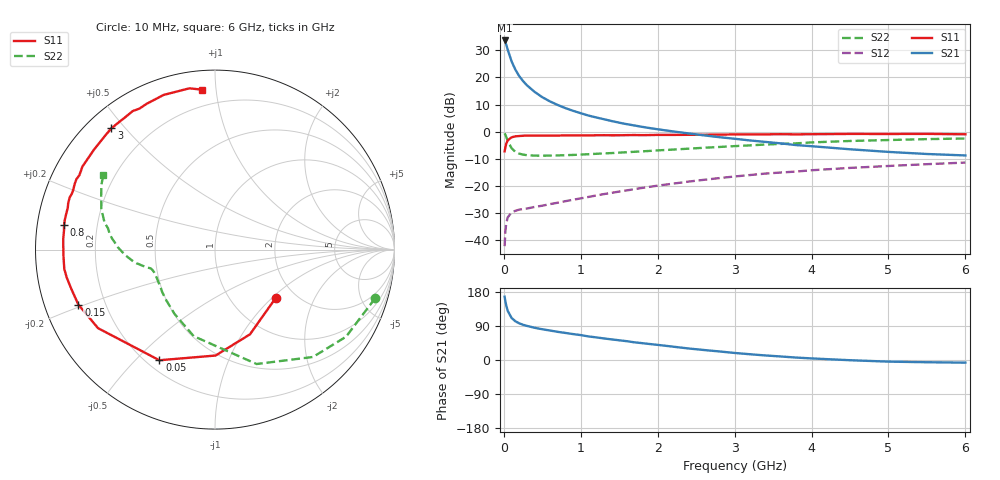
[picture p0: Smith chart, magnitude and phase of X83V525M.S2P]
! SIEMENS Small Signal Semiconductors
! BFP136W
! Si NPN RF Bipolar Junction Transistor in SOT343
! VCE = 3.5 V  IC = 25 mA
! Common Emitter S-Parameters:  September  1994
# GHz  S  MA  R  50
!  f  S11  S21  S12  S22
! GHz  MAG  ANG  MAG  ANG  MAG  ANG  MAG  ANG
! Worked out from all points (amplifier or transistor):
!   40 points, 10 MHz to 6 GHz, reference 50 ohm
!   highest |S21| = 33.7 dB at 10 MHz (marker M1)
!   |S21| within 3 dB of that: start of sweep to 46.27 MHz
!   unconditionally stable (mu >= 1): 831.5 MHz to 2.812 GHz
!   at 200 MHz: K = 0.38, MSG = 24.6 dB, |S12| = -28.8 dB
!   at 1.5 GHz: K = 1.16, MAG = 10.3 dB, |S12| = -22.1 dB
!   at 6 GHz: K = 0.97, MSG = 1.3 dB, |S12| = -11.4 dB
!   S11 on the Smith chart (normalised r, x): 10 MHz: 1.60, -1.05; 50 MHz: 0.25, -0.59; 150 MHz: 0.10, -0.19; 800 MHz: 0.08, +0.08; 3 GHz: 0.07, +0.46; 6 GHz: 0.10, +0.92
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0.01  0.4323 -38.2  48.23 167.0  0.0077 76.1  0.9325 -16.9
0.02  0.5108 -67.6  44.61 155.0  0.0144 67.2  0.8768 -33.6
0.03  0.5902 -89.7  40.99 145.0  0.0198 58.3  0.8099 -47.6
0.05  0.6901 -116.7  32.74 129.9  0.0261 44.4  0.6784 -70.0
0.1  0.785 -146.1  19.94 111.1  0.0323 31.4  0.4968 -103.8
0.15  0.8207 -158.1  13.93 102.2  0.0346 27.7  0.4232 -122.2
0.2  0.8301 -164.8  10.58 96.8  0.0364 26.7  0.3923 -133.6
0.25  0.8407 -169.4  8.576 92.9  0.0374 27.1  0.3776 -141.1
0.3  0.8466 -172.7  7.184 90.0  0.0381 27.9  0.3676 -146.3
0.4  0.8451 -177.9  5.423 85.1  0.0408 30.7  0.3612 -153.0
0.5  0.8457 178.4  4.326 81.1  0.043 33.5  0.3601 -157.1
0.6  0.8477 176.0  3.611 77.8  0.046 36.3  0.3616 -159.5
0.7  0.8478 173.0  3.111 74.3  0.0488 39.3  0.3644 -161.0
0.8  0.852 170.8  2.719 71.4  0.0521 41.6  0.3679 -162.4
1.1  0.8527 164.1  1.982 62.2  0.0624 46.8  0.3837 -164.7
1.6  0.8633 154.9  1.373 49.6  0.0825 51.4  0.4176 -167.8
2.2  0.871 144.5  1.01 35.2  0.1097 52.1  0.4668 -172.6
3  0.8888 130.5  0.74 18.6  0.1489 48.3  0.5408 178.7
3.2  0.8889 127.1  0.688 15.2  0.1582 46.8  0.5585 176.1
4.5  0.908 108.4  0.473 -0.6  0.2144 35.6  0.6732 160.2
5.5  0.9099 99.0  0.387 -5.9  0.2511 27.4  0.7283 150.4
6  0.8939 94.6  0.364 -7.0  0.2689 22.9  0.7474 146.4
